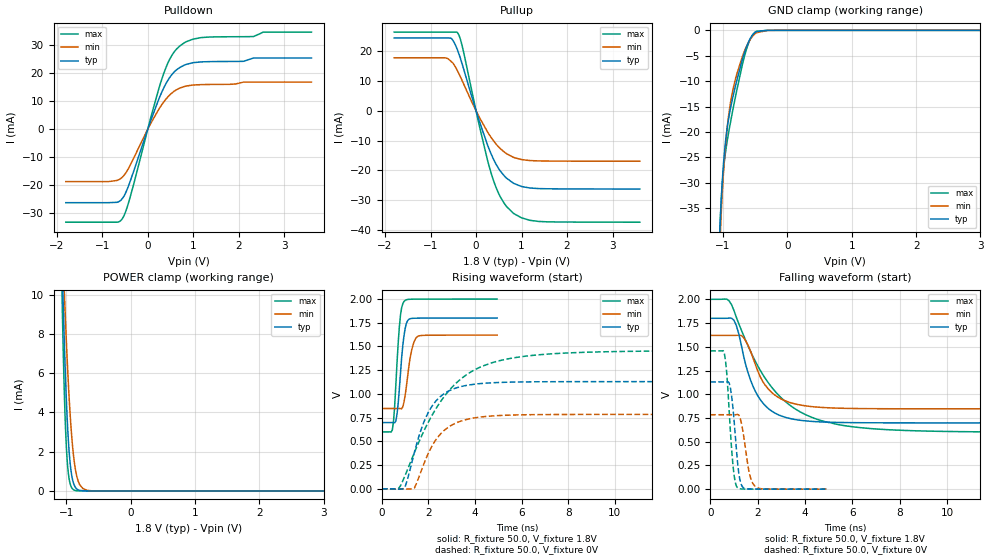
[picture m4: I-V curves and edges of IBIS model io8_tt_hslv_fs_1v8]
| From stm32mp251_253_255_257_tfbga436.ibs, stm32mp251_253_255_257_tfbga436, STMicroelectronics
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[Model]   io8_tt_hslv_fs_1v8
Model_type I/O
Polarity   Non-Inverting
Enable   Active-Low
| CAP_THRESHOLD on pad IOTT is "UDTCAPC" :
| Rising=30.0% of vddiov33m   Falling=70.0% of vddiov33m
| C_comp min and max val. don't necessarily correlate with the min and max pvt
| but are the smallest and greatest pad capacitance found.
| var   typ   min   max
C_comp   1.16098pF  1.09791pF  1.36394pF
|C_comp_pullup   764.88000fF  538.04000fF  521.01000fF
|C_comp_pulldown   396.09900fF  559.87040fF  842.92918fF
Vinl = 486.0mV
Vinh = 1.4V
Vmeas = 900.0mV   | Reference voltage for timing measurements
Cref  = 50.0pF   | Timing specification test load capacitance value
Rref  = 100.0MOhm   | Timing specification test load resistance value
Vref  = 900.0mV   | Timing specification test load voltage
[Model Spec]
| TIME_THRESHOLD on pin ZIV08M is "CMOS" :
| Rising=50.0% of vddv08m   Falling=50.0% of vddv08m
Vinl 675.70000mV 623.70000mV 735.70000mV
Vinh 1.12730V 1.01130V 1.24930V
| variable   typ   min   max
[Temperature Range] 25.0 125.0 -40.0
| variable   typ   min   max
[Voltage Range] 1.8V 1.62V 2.0V
| variable   typ   min   max
[POWER Clamp Reference] 1.8V 1.62V 2.0V
| variable   typ   min   max
[GND Clamp Reference] 0V 0V 0V
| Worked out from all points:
|   slope of the pulldown table from 0 to 0.27 V, typ, clamps not added: 22.9 ohm
|   slope of the pullup table from 0 to 0.27 V, typ, clamps not added: 22.2 ohm
|   GND clamp passes 1 mA (typ) near -0.55 V on its own axis
|   POWER clamp passes 1 mA (typ) near -0.93 V on its own axis
|   rising waveform, R_fixture 50.0, V_fixture 1.8V: 20-80 % time 227ps typ, 275ps min, 204ps max; typ from 0.698 V to 1.8 V
|   falling waveform, R_fixture 50.0, V_fixture 1.8V: 20-80 % time 929ps typ, 996ps min, 2.14ns max; typ from 1.8 V to 0.698 V
|   rising waveform, R_fixture 50.0, V_fixture 0V: 20-80 % time 1.02ns typ, 1.09ns min, 2.18ns max; typ from 0 V to 1.13 V
|   falling waveform, R_fixture 50.0, V_fixture 0V: 20-80 % time 240ps typ, 296ps min, 232ps max; typ from 1.13 V to 0 V
[POWER Clamp]
-1.8V     152.1mA    105.6mA    221.1mA
-1.07V    12.07mA    13.61mA    10.38mA
-1.05V    9.569mA    11.75mA    7.248mA
-1.03V    7.339mA    9.993mA    4.743mA
-1.01V    5.42mA     8.358mA    2.898mA
-990mV    3.841mA    6.859mA    1.662mA
-970mV    2.609mA    5.513mA    906.4uA
-940mV    1.358mA    3.806mA    344.1uA
-880mV    308.2uA    1.548mA    45.5uA
-790mV    28.46uA    298.9uA    2.106uA
-610mV    213nA      7.572uA    9.541nA
3.6V      0A         0A         0A
[GND Clamp]
-1.8V     -1.214A    -1.184A    -1.231A
-1.05V    -39.75mA   -42.57mA   -39.2mA
-1.04V    -36.64mA   -39.37mA   -36.3mA
-1.01V    -29.33mA   -31.48mA   -29.9mA
-970mV    -22.87mA   -23.87mA   -24.77mA
-920mV    -17.89mA   -17.43mA   -20.6mA
-870mV    -14.47mA   -13.19mA   -17.12mA
-790mV    -10.04mA   -8.766mA   -11.99mA
-650mV    -3.743mA   -3.579mA   -4.327mA
-570mV    -1.451mA   -1.665mA   -1.53mA
-490mV    -324.1uA   -556uA     -259.6uA
3.6V      61.92nA    2.591uA    17.99nA
| variable   typ   min   max
[Pullup Reference] 1.8V 1.62V 2.0V
| variable   typ   min   max
[Pulldown Reference] 0V 0V 0V
[Pullup]
-1.8V     24.41mA    17.74mA    26.36mA
-680mV    24.41mA    17.73mA    26.36mA
-550mV    24.31mA    16.53mA    26.36mA
-400mV    20.04mA    13.14mA    26mA
-300mV    15.41mA    9.911mA    21.43mA
70mV      -3.39mA    -2.114mA   -4.868mA
340mV     -14.76mA   -9.139mA   -21.3mA
540mV     -20.33mA   -12.79mA   -29.04mA
810mV     -24.17mA   -15.52mA   -34.21mA
1V        -25.38mA   -16.37mA   -35.89mA
1.37V     -26.08mA   -16.81mA   -37.09mA
3.6V      -26.24mA   -16.92mA   -37.35mA
[Pulldown]
-1.8V     -26.23mA   -18.7mA    -33.2mA
-680mV    -26.1mA    -18.3mA    -33.2mA
-550mV    -24.6mA    -16.98mA   -31.75mA
-400mV    -19.26mA   -13.3mA    -25.07mA
70mV      3.286mA    2.202mA    4.389mA
310mV     13.3mA     8.807mA    17.94mA
500mV     18.91mA    12.52mA    25.54mA
700mV     22.05mA    14.7mA     29.73mA
1.18V     24.11mA    15.98mA    32.81mA
2.31V     25.4mA     16.88mA    33.16mA
2.54V     25.49mA    16.88mA    34.76mA
3.6V      25.49mA    16.88mA    34.76mA
[Ramp]
dV/dt_r 677.91543mV/1.01337ns 470.52068mV/1.08941ns 874.04977mV/2.18262ns
dV/dt_f 661.10551mV/925.47757ps 464.26546mV/992.64824ps 840.45446mV/2.1443ns
R_load = 50.0
| Removed startup time: 0s 0s 0s  .
| Removed end time: 4.95ns.
[Rising Waveform]
R_fixture   = 50.0
V_fixture   = 1.8V
V_fixture_min = 1.62V
V_fixture_max = 2.0V
0s        698.3mV    846.4mV    599.4mV
450ps     698.3mV    846.4mV    620.7mV
550ps     695.9mV    846.4mV    872.9mV
650ps     785.3mV    846.3mV    1.327V
800ps     1.22V      846mV      1.832V
950ps     1.613V     914.3mV    1.975V
1.05ns    1.741V     1.073V     1.993V
1.25ns    1.795V     1.428V     1.998V
1.5ns     1.798V     1.599V     1.999V
4.95ns    1.8V       1.62V      2V
| Removed startup time: 0s 0s 0s  .
| Removed end time: 29.8ns.
[Falling Waveform]
R_fixture   = 50.0
V_fixture   = 1.8V
V_fixture_min = 1.62V
V_fixture_max = 2.0V
0s        1.8V       1.62V      2V
700ps     1.8V       1.62V      2.002V
1ns       1.78V      1.62V      1.884V
1.4ns     1.412V     1.6V       1.624V
1.8ns     1.087V     1.387V     1.399V
2.5ns     839.5mV    1.042V     1.104V
3.7ns     729.1mV    891.4mV    828mV
5.4ns     703mV      853.4mV    680.4mV
10.5ns    698.3mV    846.4mV    606.1mV
29.8ns    698.3mV    846.4mV    599.4mV
| Removed startup time: 0s 0s 0s  .
| Removed end time: 29.9ns.
[Rising Waveform]
R_fixture   = 50.0
V_fixture   = 0V
V_fixture_min = 0V
V_fixture_max = 0V
0s        0V         0V         0V
700ps     -3.033mV   -8.996uV   -1.285mV
1ns       21.36mV    -2.045mV   141.5mV
1.4ns     387.1mV    9.823mV    383.8mV
1.8ns     701mV      260.5mV    606.8mV
2.5ns     969.9mV    573.1mV    912.2mV
3.7ns     1.093V     734.4mV    1.213V
5.4ns     1.124V     775.9mV    1.369V
10.6ns    1.13V      784mV      1.449V
29.9ns    1.13V      784.1mV    1.457V
| Removed startup time: 0s 0s 0s  .
| Removed end time: 4.9ns.
[Falling Waveform]
R_fixture   = 50.0
V_fixture   = 0V
V_fixture_min = 0V
V_fixture_max = 0V
0s        1.13V      784.1mV    1.457V
600ps     1.13V      784.1mV    1.425V
700ps     1.13V      784.1mV    1.217V
850ps     1.07V      784.1mV    618.7mV
1ns       745.4mV    783.9mV    161.4mV
1.15ns    291.9mV    786.9mV    15.84mV
1.35ns    28.83mV    654.1mV    1.956mV
1.65ns    1.582mV    170.8mV    799.4uV
1.9ns     799.6uV    29.27mV    499.8uV
4.9ns     0V         0V         0V
